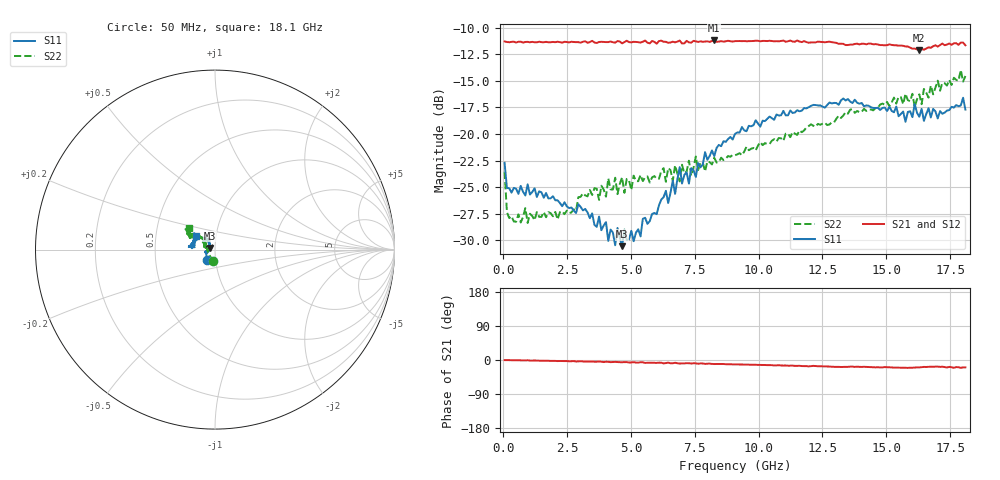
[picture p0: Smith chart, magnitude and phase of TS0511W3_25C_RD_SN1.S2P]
! Network Analyzer HP8720D.06.14 Serial No. US36140669
! 17 Jun 2005  08:05:30
! Frequency  S11  S21  S12  S22
# HZ  S  DB R 50
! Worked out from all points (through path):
!   201 points, 50 MHz to 18.1 GHz, reference 50 ohm
!   highest |S21| = -11.19 dB at 8.263 GHz (marker M1); lowest = -12.1 dB at 16.3 GHz (marker M2)
!   group delay of S21, straight-line fit = 3.36 ps
!   lowest |S11| = -30.6 dB at 4.653 GHz (marker M3), VSWR 1.06, Z = 47.2 + j0.818 ohm
!   |S11| at or under -10 dB: start of sweep to end of sweep
!   |S22| runs from -28.4 to -14.0 dB; largest |S21 - S12| = 0.0072
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5e7  -22.70 -127.8  -11.28 -0.3  -11.30 -0.1  -23.56 -98.6
1.4025e8  -25.08 -150.5  -11.33 -0.3  -11.35 -0.2  -27.35 -140.3
4.11e8  -25.07 -166.2  -11.31 -0.6  -11.35 -0.5  -28.24 -164.6
2.12575e9  -26.24 -164.5  -11.30 -2.9  -11.36 -2.7  -28.04 164.5
3.1185e9  -27.19 -166.0  -11.31 -3.9  -11.35 -3.9  -25.57 167.5
4.382e9  -30.47 175.1  -11.39 -4.9  -11.31 -5.4  -24.11 163.3
4.47225e9  -28.85 169.0  -11.25 -5.4  -11.33 -5.0  -25.66 166.3
4.65275e9  -30.56 163.0  -11.46 -5.8  -11.32 -5.5  -24.07 166.1
4.743e9  -28.99 165.9  -11.34 -5.5  -11.39 -5.5  -25.54 161.5
5.37475e9  -29.64 147.6  -11.38 -5.7  -11.27 -6.0  -23.86 157.1
6.09675e9  -26.71 132.7  -11.25 -7.0  -11.21 -7.2  -24.21 155.5
6.7285e9  -25.63 130.9  -11.37 -7.3  -11.44 -8.0  -22.94 149.4
6.909e9  -23.11 126.7  -11.20 -9.3  -11.34 -9.0  -24.46 145.3
7.27e9  -24.67 123.8  -11.37 -8.4  -11.36 -9.3  -22.51 147.7
7.36025e9  -23.21 121.4  -11.39 -9.2  -11.37 -8.6  -23.93 150.5
7.54075e9  -24.04 122.2  -11.28 -8.8  -11.18 -9.7  -22.10 149.9
8.26275e9  -22.08 132.8  -11.19 -10.7  -11.25 -10.8  -22.24 138.8
9.075e9  -19.98 137.9  -11.25 -11.5  -11.25 -11.4  -22.00 139.7
1.21435e10  -17.26 167.8  -11.37 -15.5  -11.35 -15.7  -19.22 140.0
1.512175e10  -17.44 172.7  -11.55 -19.2  -11.54 -18.8  -17.37 148.2
1.6295e10  -18.37 161.7  -12.07 -19.6  -11.96 -19.5  -16.26 154.0
1.81e10  -17.70 143.6  -11.64 -19.6  -11.69 -21.0  -14.54 139.6
